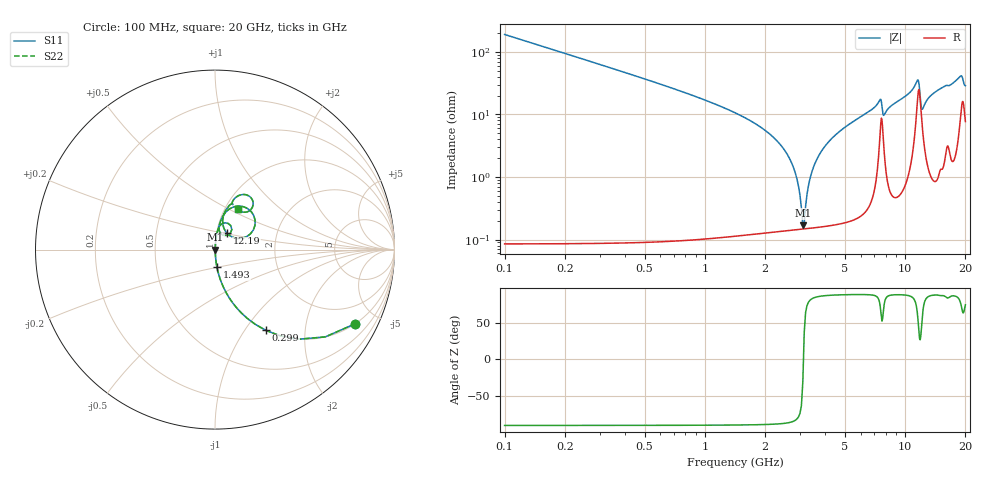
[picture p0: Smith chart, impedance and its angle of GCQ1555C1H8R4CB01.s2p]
!Murata Part Number: GCQ1555C1H8R4CB01
!These Parameters are Measured in Series Mode Connection
!Data Generated on Mar 13, 2026
!  o--ll--o
!Port1  Port2
!  o------o
!Operation Temp=25[degC], DC Bias Voltage=0[V]
!Freq. Start=100[MHz] Stop=20[GHz] 401[Steps]
# Hz S RI R 50
!Freq.(Hz) S11(Real) S11(Imag) S21(Real) S21(Imag) S12(Real) S12(Imag) S22(Real) S22(Imag)
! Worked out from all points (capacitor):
!   401 points, 100 MHz to 20 GHz, reference 50 ohm
!   read as one part in series: C = 8.4 pF near 199.5 MHz
!   lowest |Z| = 170 mohm at 3.085 GHz (marker M1)
!   series resonance near 3.107 GHz, so ESL is about 310 pH
!   S11 on the Smith chart (normalised r, x): 100 MHz: 1.00, -3.79; 299 MHz: 1.00, -1.26; 1.493 GHz: 1.00, -0.20; 12.19 GHz: 1.12, +0.21; 20 GHz: 1.15, +0.55
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1e8  0.7817 -0.4129  0.2183 0.4129  0.2183 0.4129  0.7817 -0.4129
2.99e8  0.283 -0.4498  0.717 0.4498  0.717 0.4498  0.283 -0.4498
6.4725e8  0.0734 -0.2592  0.9266 0.2592  0.9266 0.2592  0.0734 -0.2592
1.493e9  0.0106 -0.0965  0.9894 0.0965  0.9894 0.0965  0.0106 -0.0965
2.5875e9  0.00189 -0.0224  0.9981 0.0224  0.9981 0.0224  0.00189 -0.0224
2.83625e9  0.00155 -0.0111  0.9985 0.0111  0.9985 0.0111  0.00155 -0.0111
3.085e9  0.00147 -0.000856  0.9985 0.000856  0.9985 0.000856  0.00147 -0.000856
3.1845e9  0.00149 0.00303  0.9985 -0.00303  0.9985 -0.00303  0.00149 0.00303
3.43325e9  0.00167 0.0123  0.9983 -0.0123  0.9983 -0.0123  0.00167 0.0123
3.83125e9  0.00227 0.026  0.9977 -0.026  0.9977 -0.026  0.00227 0.026
4.42825e9  0.00372 0.0448  0.9963 -0.0448  0.9963 -0.0448  0.00372 0.0448
6.7665e9  0.0174 0.1148  0.9826 -0.1148  0.9826 -0.1148  0.0174 0.1148
7.51275e9  0.0736 0.1456  0.9264 -0.1456  0.9264 -0.1456  0.0736 0.1456
7.861e9  0.0328 0.0897  0.9672 -0.0897  0.9672 -0.0897  0.0328 0.0897
1.005e10  0.0437 0.1859  0.9563 -0.1859  0.9563 -0.1859  0.0437 0.1859
1.15425e10  0.204 0.2088  0.796 -0.2088  0.796 -0.2088  0.204 0.2088
1.189075e10  0.1528 0.0635  0.8472 -0.0635  0.8472 -0.0635  0.1528 0.0635
1.218925e10  0.0676 0.0908  0.9324 -0.0908  0.9324 -0.0908  0.0676 0.0908
1.338325e10  0.0466 0.1858  0.9534 -0.1858  0.9534 -0.1858  0.0466 0.1858
1.67165e10  0.0957 0.2567  0.9043 -0.2567  0.9043 -0.2567  0.0957 0.2567
1.89055e10  0.1912 0.2971  0.8088 -0.2971  0.8088 -0.2971  0.1912 0.2971
2e10  0.1292 0.2242  0.8708 -0.2242  0.8708 -0.2242  0.1292 0.2242
